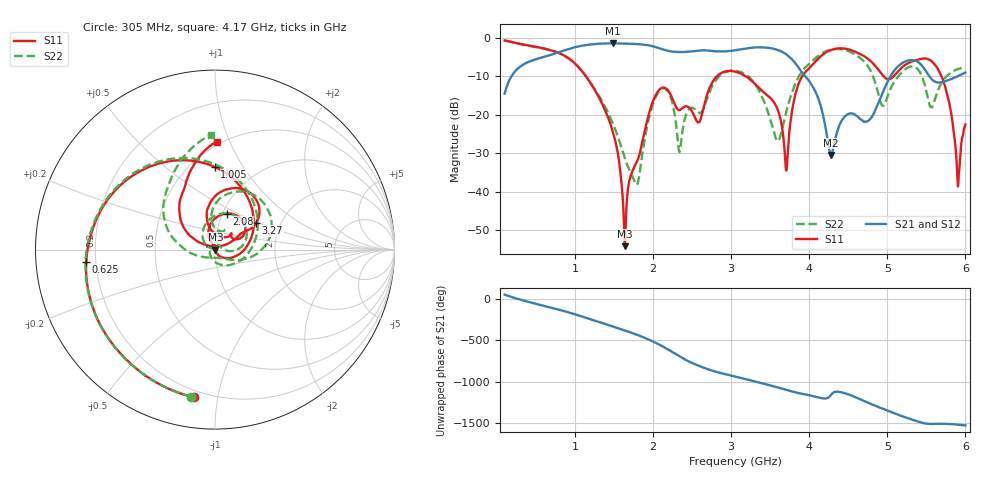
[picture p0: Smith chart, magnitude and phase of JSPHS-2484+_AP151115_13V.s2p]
!Mini-Circuits Laboratory
!S-Parameters
!Run/Lot/Date Code:MF33450/NA/1551
!Fixture/SN/Due: 90-4-20-21/70546/03/17/16
!Connection:PORT<IN> - pin<1>; PORT<OUT> - pin<7>;PORT<BIAS> - pin<4>;
!Tested With:PORT EXTENTION
!Network Analyzer:AG E5071C/74883/05/12/16
!Created: 01-07-2016 at 14:11:09
!MODEL: JSPHS-2484+
!S/N: V=13V
# MHZ S DB R 50
!Frequency  S11 dB  S11 DEG  S21 dB  S21 DEG  S12 dB  S12 DEG  S22 dB  S22 DEG
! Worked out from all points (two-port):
!   1181 points, 100 MHz to 6 GHz, reference 50 ohm
!   highest |S21| = -1.42 dB at 1.49 GHz (marker M1); lowest = -30.5 dB at 4.28 GHz (marker M2)
!   |S21| within 3 dB of the highest: 691.5 MHz to 3.716 GHz (3.024 GHz wide, 137 % of centre)
!   lowest |S11| = -54.2 dB at 1.64 GHz (marker M3), VSWR 1.00, Z = 50.2 + j0.0235 ohm
!   |S11| at or under -10 dB: 1.141 GHz to 2.817 GHz (1.676 GHz wide, 84.7 % of centre); 3.188 GHz to 3.91 GHz (722.5 MHz wide, 20.4 % of centre); 5.692 GHz to end of sweep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
!   |S22| runs from -38.2 to -0.7 dB; largest |S21 - S12| = 0.0052
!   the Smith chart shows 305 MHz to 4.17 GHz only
!   S11 on the Smith chart (normalised r, x): 305 MHz: 0.16, -0.85; 625 MHz: 0.16, -0.05; 1.005 GHz: 0.65, +0.76; 2.08 GHz: 1.04, +0.44; 3.27 GHz: 1.50, +0.48; 4.17 GHz: 0.47, +0.90
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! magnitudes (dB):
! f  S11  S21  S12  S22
! 100 MHz  -0.7  -14.5  -14.5  -0.7
! 305 MHz  -1.6  -7.4  -7.4  -1.6
! 625 MHz  -2.8  -4.8  -4.8  -2.9
! 1.005 GHz  -6.7  -2.4  -2.4  -6.8
! 1.085 GHz  -8.5  -2.0  -2.0  -8.5
! 1.49 GHz  -24.8  -1.4  -1.4  -22.5
! 1.64 GHz  -54.2  -1.5  -1.5  -31.3
! 1.8 GHz  -31.9  -1.6  -1.6  -38.0
! 2.07 GHz  -13.7  -2.6  -2.6  -14.1
! 2.08 GHz  -13.5  -2.7  -2.7  -13.8
! 2.34 GHz  -18.8  -3.7  -3.7  -29.7
! 3.05 GHz  -8.8  -3.2  -3.2  -8.5
! 3.27 GHz  -11.3  -2.5  -2.6  -11.1
! 3.59 GHz  -18.3  -3.1  -3.1  -26.8
! 3.705 GHz  -34.5  -4.3  -4.3  -19.3
! 4.035 GHz  -7.1  -12.3  -12.3  -6.1
! 4.17 GHz  -4.4  -19.5  -19.5  -3.9
! 4.28 GHz  -3.2  -30.5  -30.4  -3.0
! 5.02 GHz  -10.8  -10.8  -10.8  -14.3
! 5.615 GHz  -7.1  -11.4  -11.4  -15.7
! 5.91 GHz  -37.8  -9.9  -9.9  -8.1
! 6 GHz  -22.5  -9.0  -9.0  -7.6
